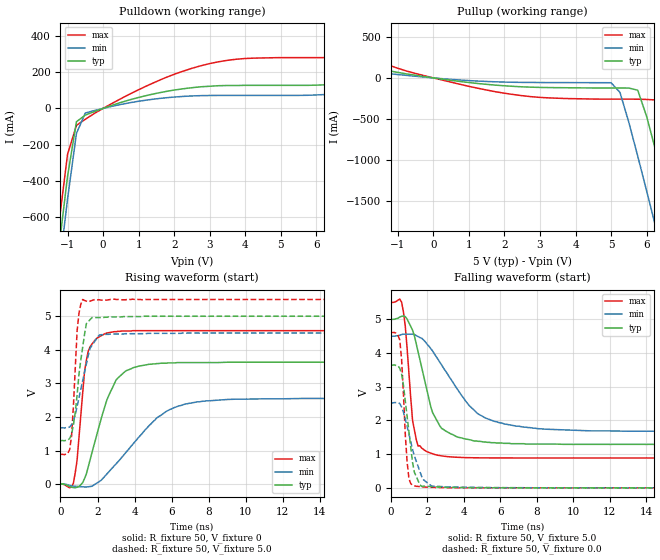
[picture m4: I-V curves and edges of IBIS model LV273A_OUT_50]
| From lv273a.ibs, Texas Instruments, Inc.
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|   Model LV273A_OUT_50
[Model]   LV273A_OUT_50
Model_type  Output
Polarity   Non-Inverting
Vmeas = 2.50v
Cref = 15pf
| variable   typ   min   max
C_comp   7.60pf   5.70pf   9.50pf
[Temperature Range]   25   85   -40
[Voltage Range]   5.0   4.5   5.5
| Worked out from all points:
|   slope of the pulldown table from 0 to 0.75 V, typ, clamps not added: 15.9 ohm
|   slope of the pullup table from 0 to 0.75 V, typ, clamps not added: 17.2 ohm
|   rising waveform, R_fixture 50, V_fixture 0: 20-80 % time 1.24ns typ, 2.55ns min, 461ps max; typ from 0 V to 3.63 V
|   falling waveform, R_fixture 50, V_fixture 5.0: 20-80 % time 1.09ns typ, 2.25ns min, 433ps max; typ from 5 V to 1.29 V
|   rising waveform, R_fixture 50, V_fixture 5.0: 20-80 % time 475ps typ, 680ps min, 259ps max; typ from 1.29 V to 5 V
|   falling waveform, R_fixture 50, V_fixture 0.0: 20-80 % time 478ps typ, 781ps min, 271ps max; typ from 3.64 V to 0 V
[Pulldown]
|   Voltage   I(typ)   I(min)   I(max)
-5V       -7.35A     -7.47A     -7.23A
-1.25V    -781mA     -909mA     -646mA
-1V       -374mA     -499mA     -253mA
-750mV    -73.6mA    -138mA     -93.5mA
-500mV    -37mA      -25.4mA    -60mA
1.25V     72.2mA     46.5mA     126mA
2.75V     119mA      70.2mA     235mA
4V        127mA      71.2mA     275mA
6.25V     130mA      76.4mA     280mA
7.25V     148mA      90.2mA     300mA
8.5V      184mA      114mA      355mA
10V       236mA      145mA      444mA
[Pullup]
|   Voltage   I(typ)   I(min)   I(max)
-5V       318mA      174mA      597mA
1.5V      -78.8mA    -43.5mA    -148mA
5V        -123mA     -58.9mA    -259mA
5.25V     -123mA     -177mA     -259mA
5.75V     -150mA     -956mA     -260mA
6V        -471mA     -1.38A     -263mA
6.25V     -880mA     -1.81A     -269mA
6.5V      -1.3A      -2.24A     -452mA
6.75V     -1.74A     -2.68A     -855mA
7.25V     -2.61A     -3.55A     -1.71A
7.5V      -3.04A     -3.99A     -2.15A
10V       -7.45A     -8.4A      -6.56A
[Ramp]
| variable   typ   min   max
dV/dt_r   2.18E+00/1.19E-09   1.53E+00/2.53E-09   2.78E+00/4.81E-10
dV/dt_f   2.29E+00/1.07E-09   1.74E+00/2.28E-09   2.83E+00/4.19E-10
R_load = 50
[Rising Waveform]
R_fixture = 50
V_fixture = 0
|   Time   V(typ)   V(min)   V(max)
0s        0V         0V         0V
700ps     -104mV     -61.5mV    26.8mV
900ps     -94.7mV    -70.8mV    723mV
1.3ns     165mV      -85.5mV    3.36V
1.5ns     514mV      -80.7mV    3.96V
2.5ns     2.5V       297mV      4.5V
3.6ns     3.39V      986mV      4.56V
5.2ns     3.59V      1.97V      4.57V
6.7ns     3.62V      2.38V      4.57V
25ns      3.63V      2.55V      4.57V
[Falling Waveform]
R_fixture = 50
V_fixture = 5.0
V_fixture_min = 4.5
V_fixture_max = 5.5
|   Time   V(typ)   V(min)   V(max)
0s        5V         4.5V       5.5V
600ps     5.09V      4.55V      5.51V
800ps     5.08V      4.56V      4.81V
1.2ns     4.68V      4.56V      2V
1.5ns     4.04V      4.49V      1.24V
2.4ns     2.13V      3.97V      991mV
2.8ns     1.76V      3.64V      947mV
4.3ns     1.43V      2.44V      895mV
6.2ns     1.32V      1.9V       887mV
25ns      1.29V      1.67V      886mV
[Rising Waveform]
R_fixture = 50
V_fixture = 5.0
V_fixture_min = 4.5
V_fixture_max = 5.5
|   Time   V(typ)   V(min)   V(max)
0s        1.29V      1.67V      886mV
500ps     1.36V      1.7V       1.03V
600ps     1.49V      1.77V      1.44V
700ps     1.76V      1.89V      2.32V
900ps     2.66V      2.32V      4.57V
1.2ns     4.08V      3.08V      5.5V
1.4ns     4.78V      3.58V      5.45V
1.6ns     4.9V       4.05V      5.45V
2.2ns     4.96V      4.45V      5.48V
25ns      5V         4.5V       5.5V
[Falling Waveform]
R_fixture = 50
V_fixture = 0.0
|   Time   V(typ)   V(min)   V(max)
0s        3.64V      2.53V      4.61V
500ps     3.55V      2.5V       4.39V
600ps     3.38V      2.4V       3.81V
800ps     2.59V      2.04V      1.6V
900ps     2.13V      1.83V      786mV
1ns       1.67V      1.6V       274mV
1.3ns     461mV      945mV      59.6mV
1.8ns     52.8mV     239mV      25.5mV
2.3ns     34.4mV     47.9mV     12.9mV
25ns      0V         0V         6.64uV
